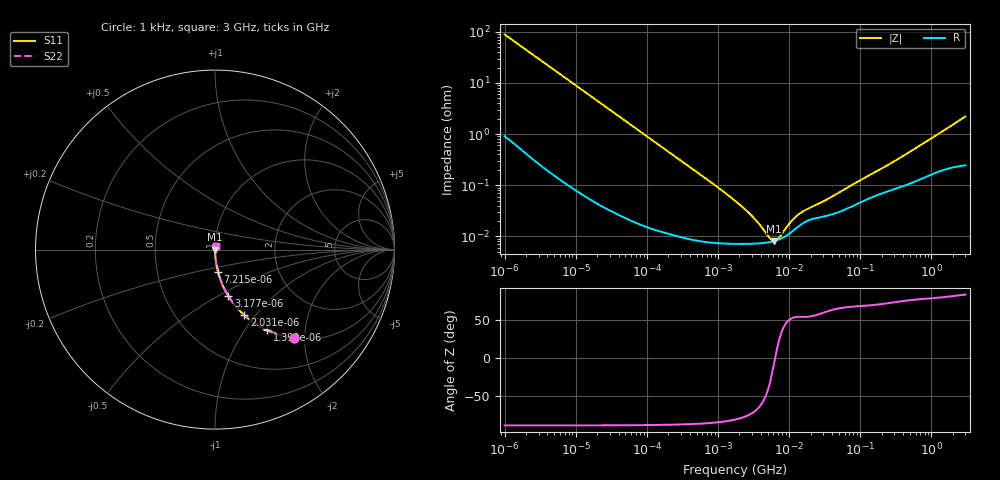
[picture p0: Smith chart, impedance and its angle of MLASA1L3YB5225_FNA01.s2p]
! MLASA1L3YB5225_FNA01  S-PARAMETER MODEL  ( Standard Model )
! Model Generated by TAIYO YUDEN Corporation (http://www.ty-top.com)
! Version 1.0
! TAIYO YUDEN Control No. 220601
! Copyright(c) 2013 TAIYO YUDEN CO.,LTD. All Rights Reserved.
! Product Description (link to TY-COMPAS)
! https://ds.yuden.co.jp/TYCOMPAS/or/detail?pn=MLASA1L3YB5225MFNA01&u=M
! Products Name : Multilayer Ceramic Capacitors
! Characteristics :
!  Capacitance : 2.2 [uF] , Rated Voltage : 4 [V] , TCC : X5R
!  Case Size : 1.0 x 0.5 / 0.039 x 0.02 [mm/inch] , Thickness : 0.3 / 0.012 [mm/inch]
!  (Conditions: Temperature = 25 [degC] , DC Bias Voltage = 0 [V])
! External Node Assignments :
!  1  o---| |---o  2
! GND o---------o GND
! Frequency Range : 1kHz  -  3GHz  [ 401 STEP ]
# MHZ S RI R 50
! Freq[MHz].  S11 Real  S11 Imag  S21 Real  S21 Imag  S12 Real  S12 Imag  S22 Real  S22 Imag
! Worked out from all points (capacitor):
!   401 points, 1 kHz to 3 GHz, reference 50 ohm
!   read as one part in series: C = 1.79 uF near 1.077 kHz
!   lowest |Z| = 8.15 mohm at 6.153 MHz (marker M1)
!   series resonance near 6.356 MHz, so ESL is about 350 pH
!   S11 on the Smith chart (normalised r, x): 1 kHz: 1.02, -1.77; 1.399 kHz: 1.01, -1.27; 2.031 kHz: 1.01, -0.88; 3.177 kHz: 1.00, -0.56; 7.215 kHz: 1.00, -0.25; 3 GHz: 1.00, +0.04
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0.001  0.4407 -0.4914  0.5593 0.4914  0.5593 0.4914  0.4407 -0.4914
0.001399  0.2896 -0.4486  0.7104 0.4486  0.7104 0.4486  0.2896 -0.4486
0.002031  0.1637 -0.3654  0.8363 0.3654  0.8363 0.3654  0.1637 -0.3654
0.003177  0.0752 -0.2594  0.9248 0.2594  0.9248 0.2594  0.0752 -0.2594
0.007215  0.0162 -0.1221  0.9838 0.1221  0.9838 0.1221  0.0162 -0.1221
0.01216  0.00609 -0.0734  0.9939 0.0734  0.9939 0.0734  0.00609 -0.0734
0.033275  0.00103 -0.0271  0.999 0.0271  0.999 0.0271  0.00103 -0.0271
0.147855  0.000165 -0.00616  0.9998 0.00616  0.9998 0.00616  0.000165 -0.00616
0.762639  7.74e-05 -0.00119  0.9999 0.00119  0.9999 0.00119  7.74e-05 -0.00119
1.732051  7.17e-05 -0.000494  0.9999 0.000494  0.9999 0.000494  7.17e-05 -0.000494
3.03007  7.2e-05 -0.000237  0.9999 0.000237  0.9999 0.000237  7.2e-05 -0.000237
4.919932  7.6e-05 -7.62e-05  0.9999 7.62e-05  0.9999 7.62e-05  7.6e-05 -7.62e-05
5.502215  7.81e-05 -4.27e-05  0.9999 4.27e-05  0.9999 4.27e-05  7.81e-05 -4.27e-05
6.153411  8.09e-05 -9.55e-06  0.9999 9.55e-06  0.9999 9.55e-06  8.09e-05 -9.55e-06
7.414467  8.84e-05 4.57e-05  0.9999 -4.57e-05  0.9999 -4.57e-05  8.84e-05 4.57e-05
10.37087  0.000117 0.000146  0.9999 -0.000146  0.9999 -0.000146  0.000117 0.000146
12.49624  0.000144 0.000198  0.9999 -0.000198  0.9999 -0.000198  0.000144 0.000198
15.62917  0.000181 0.00025  0.9998 -0.00025  0.9998 -0.00025  0.000181 0.00025
21.06097  0.000218 0.000312  0.9998 -0.000312  0.9998 -0.000312  0.000218 0.000312
34.19675  0.000254 0.000465  0.9997 -0.000465  0.9997 -0.000465  0.000254 0.000465
256.0921  0.000784 0.00246  0.9992 -0.00246  0.9992 -0.00246  0.000784 0.00246
3000  0.00293 0.0219  0.9971 -0.0219  0.9971 -0.0219  0.00293 0.0219
